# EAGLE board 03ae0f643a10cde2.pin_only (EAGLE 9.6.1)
REV: B

Size 17.78 x 25.4 mm. Coordinates in mm from the lower left corner, seen from the top.
Outline: 2.54,0 15.24,0 arc90 17.78,2.54 17.78,22.86 arc90 15.24,25.4 2.54,25.4 arc90 0,22.86 0,2.54 arc90 2.54,0
Copper layers (1*16): Top 0.035mm / dielectric 1.5mm / Bottom 0.035mm
Design rules "adafruit *": minimum track width 8mil, minimum drill 15.5mil, track to track 8mil, track to pad 8mil, pad to pad 8mil, via to via 8mil, smd to smd 8mil, copper to edge 10mil, drill to drill 8mil, minimum pad ring 10mil, minimum via ring 8mil, stop-mask expansion 2mil, vias tented up to drill 20mil, thermal gap 10mil
Net classes: 1 highpower: width 0.406 mm, drill 0.483 mm; 2 lowpower: width 0.305 mm, drill 0.483 mm

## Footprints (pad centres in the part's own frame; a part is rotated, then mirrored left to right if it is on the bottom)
0603-NO = smd 1.075 x 1: 1 -0.85,0; 2 0.85,0
0805-NO = smd 1.24 x 1.5: 1 -0.95,0; 2 0.95,0
JST_SH4 = smd 0.6 x 1.55: 1 -1.5,2.514; 2 -0.5,2.514; 3 0.5,2.514; 4 1.5,2.514 | smd 1.2 x 1.8: MT1 -2.8,-1.386; MT2 2.8,-1.386
CHIPLED_0603_NOOUTLINE = smd 0.8 x 0.8: A 0,-0.75; C 0,0.75
SOD-323 = smd 1.35 x 0.8: A 1.27,0; C -1.27,0
FIDUCIAL_1MM = smd 1 x 1: 1 0,0
1X06_ROUND_70 = drill 1 pad 1.778: 1 -6.35,0; 2 -3.81,0; 3 -1.27,0; 4 1.27,0; 5 3.81,0; 6 6.35,0
SOT363 = smd 0.5 x 0.5: 1 -0.75,-0.9; 3 0.75,-0.9; 4 0.75,0.9; 6 -0.75,0.9 | smd 0.4 x 0.5: 2 0,-0.9; 5 0,0.9
RESPACK_4X0603 = smd 0.45 x 0.9: 1 -1.3,-0.85; 2 -0.4,-0.85; 3 0.4,-0.85; 4 1.3,-0.85; 5 1.3,0.85; 6 0.4,0.85; 7 -0.4,0.85; 8 -1.3,0.85
SOLDERJUMPER_ARROW_NOPASTE = smd 0.762 x 1.524: 1 -1.016,0; 2 1.016,0
LGA16_3X3MM = smd 0.5 x 0.25: 1 -1.35,1; 2 -1.35,0.5; 3 -1.35,0; 4 -1.35,-0.5; 5 -1.35,-1; 9 1.35,-1; 10 1.35,-0.5; 11 1.35,0; 12 1.35,0.5; 13 1.35,1 | smd 0.25 x 0.5: 6 -0.5,-1.35; 7 0,-1.35; 8 0.5,-1.35; 14 0.5,1.35; 15 0,1.35; 16 -0.5,1.35
SOT23-5 = smd 0.55 x 1.2: 1 -0.95,-1.3; 2 0,-1.3; 3 0.95,-1.3; 4 0.95,1.3; 5 -0.95,1.3
MOUNTINGHOLE_2.5_PLATED = drill 2.5 pad 3.2: P$1 0,0

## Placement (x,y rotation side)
C1  0.1uF  [0603-NO]  5.4,5.52 180 top
C2  10uF  [0805-NO]  12.32,7.49 90 top
C3  10uF  [0805-NO]  12.51,10.99 270 top
CONN3  STEMMA_I2C_QT  [JST_SH4]  8.89,22.86 180 top
CONN4  STEMMA_I2C_QT  [JST_SH4]  8.89,2.54 0 top
D1  GREEN  [CHIPLED_0603_NOOUTLINE]  5.21,3.56 180 top
D2  1N4148  [SOD-323]  6.03,12.95 270 top
FID3  FIDUCIAL_1MM  [FIDUCIAL_1MM]  12.7,4.83 90 top
FID4  FIDUCIAL_1MM  [FIDUCIAL_1MM]  4.32,20 90 top
JP2  [1X06_ROUND_70]  2.54,12.7 270 top
JP3  [1X06_ROUND_70]  15.24,12.7 90 top
Q2  BSS138  [SOT363]  10.03,16.89 180 top
R1  10K  [RESPACK_4X0603]  5.84,8.26 270 top
R3  10K  [RESPACK_4X0603]  6.6,17.14 270 top
SJ1  [SOLDERJUMPER_ARROW_NOPASTE]  6.03,17.02 90 bottom
U1  LIS3DHTR  [LGA16_3X3MM]  8.89,12.7 270 top
U2  AP2112K-3.3  [SOT23-5]  9.4,7.87 90 top
U$1  MOUNTINGHOLE2.5  [MOUNTINGHOLE_2.5_PLATED]  2.54,2.54 90 top
U$12  [ADAFRUIT_2.5MM]  13.72,15.05 90 top
U$17  MOUNTINGHOLE2.5  [MOUNTINGHOLE_2.5_PLATED]  2.54,22.86 90 top
U$19  MOUNTINGHOLE2.5  [MOUNTINGHOLE_2.5_PLATED]  15.24,2.54 90 top
U$21  MOUNTINGHOLE2.5  [MOUNTINGHOLE_2.5_PLATED]  15.24,22.86 90 top
U$25  [PCBFEAT-REV-040]  12.76,21.02 270 bottom
U$30  [STEMMAQT]  13.34,22.48 0 bottom
U$31  [STEMMAQT]  4.45,2.92 180 bottom

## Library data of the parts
C1-C3 CONN3 CONN4 D1 D2 JP2 JP3 Q2 R1 R3 U1 U2 U$12 U$25 = microbuilder
FID3 FID4 SJ1 U$1 U$17 U$19 U$21 = microbuilder; BOM: EXCLUDE
U$30 U$31 = silks

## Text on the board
tPlace: X | CS | Z | INT | Y | SDO | SDA | LIS3DH | A1 | SCL | A2 | GND | A3 | 3Vo | I2 | VIN | on
bPlace: addr | LIS3DH | 3-axis Accelerometer / ±2g/±4g/±8g / I2C addr 0x18 | VLogic/Vcc: 3-5VDC

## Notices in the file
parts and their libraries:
microbuilder: This work is placed in the public domain, and may be freely used for commercial and non-commercial work with the following conditions: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
